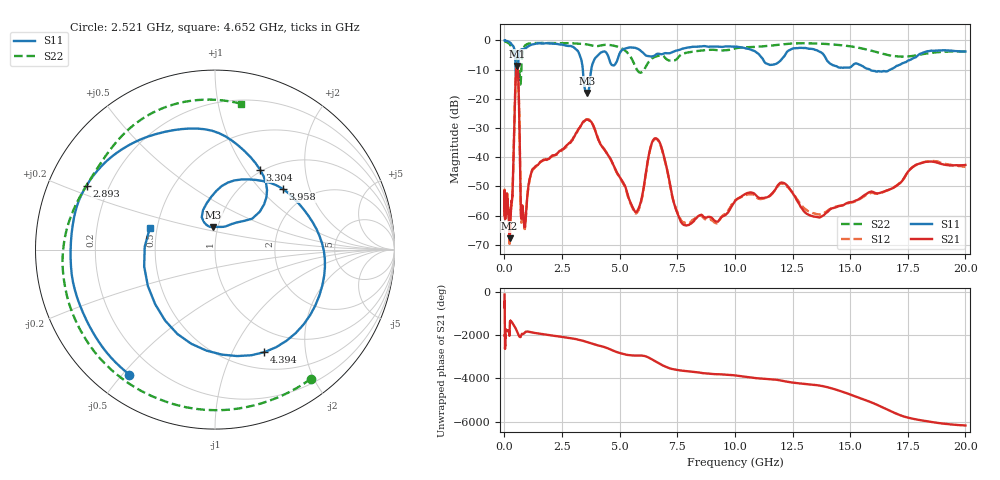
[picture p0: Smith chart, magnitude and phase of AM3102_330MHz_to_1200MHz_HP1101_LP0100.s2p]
! Date/Time: Tue, Sep 11, 2018 5:22 PM
! Network Analyzer: Agilent Technologies E8362B Rev: A.07.50.63
! Sweep from 0.010 to 20.000 GHz, 1601 Points, Sweep Type: LOG
! Power Supply: 4.949 V, 0.001 A
# Hz S DB R 50
!freq MagS11 AngS11 MagS21 AngS21 MagS12 AngS12 MagS22 AngS22
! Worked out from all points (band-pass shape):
!   1601 points, 10 MHz to 20 GHz, reference 50 ohm
!   highest |S21| = -8.72 dB at 553.8 MHz (marker M1); lowest = -67.8 dB at 223.5 MHz (marker M2)
!   |S21| within 3 dB of the highest: 497.8 MHz to 595.1 MHz (97.29 MHz wide, 17.8 % of centre)
!   lowest |S11| = -18.0 dB at 3.599 GHz (marker M3), VSWR 1.29, Z = 47.6 + j12.1 ohm
!   |S11| at or under -10 dB: 486.8 MHz to 566 MHz (79.14 MHz wide, 15 % of centre); 3.403 GHz to 3.768 GHz (365.6 MHz wide, 10.2 % of centre); 15.86 GHz to 16.74 GHz (884 MHz wide, 5.42 % of centre)
!   |S22| runs from -15.1 to -0.2 dB; largest |S21 - S12| = 0.0052
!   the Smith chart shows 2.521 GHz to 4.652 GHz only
!   S11 on the Smith chart (normalised r, x): 2.521 GHz: 0.11, -0.52; 2.893 GHz: 0.12, +0.23; 3.304 GHz: 0.97, +1.17; 3.958 GHz: 1.48, +1.35; 4.394 GHz: 0.70, -1.34; 4.652 GHz: 0.46, +0.13
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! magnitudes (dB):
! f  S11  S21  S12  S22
! 10 MHz  0.0  -54.2  -55.6  -0.2
! 35.55 MHz  -0.1  -61.2  -59.2  -0.3
! 126.4 MHz  -0.2  -55.1  -53.5  -0.7
! 223.5 MHz  -0.7  -67.8  -69.8  -1.2
! 351 MHz  -1.6  -52.6  -52.8  -3.9
! 447.2 MHz  -3.6  -23.7  -23.7  -4.1
! 553.8 MHz  -10.5  -8.7  -8.8  -10.2
! 623.6 MHz  -5.4  -18.4  -18.4  -10.3
! 733 MHz  -3.1  -60.9  -62.3  -10.2
! 1.59 GHz  -1.0  -41.5  -41.4  -0.9
! 2.521 GHz  -1.5  -37.3  -37.4  -1.0
! 2.893 GHz  -1.9  -34.7  -34.5  -1.0
! 3.304 GHz  -5.8  -29.4  -29.4  -1.1
! 3.599 GHz  -18.0  -27.2  -27.0  -1.4
! 3.958 GHz  -5.9  -31.4  -31.3  -2.0
! 4.394 GHz  -4.0  -38.1  -38.0  -1.5
! 4.652 GHz  -8.3  -41.4  -41.5  -1.7
! 5.652 GHz  -2.5  -58.5  -59.0  -8.4
! 6.549 GHz  -5.0  -33.5  -33.7  -5.6
! 7.92 GHz  -2.5  -63.4  -62.6  -4.2
! 13.61 GHz  -3.6  -60.6  -59.6  -1.1
! 20 GHz  -3.8  -42.7  -43.3  -3.8
